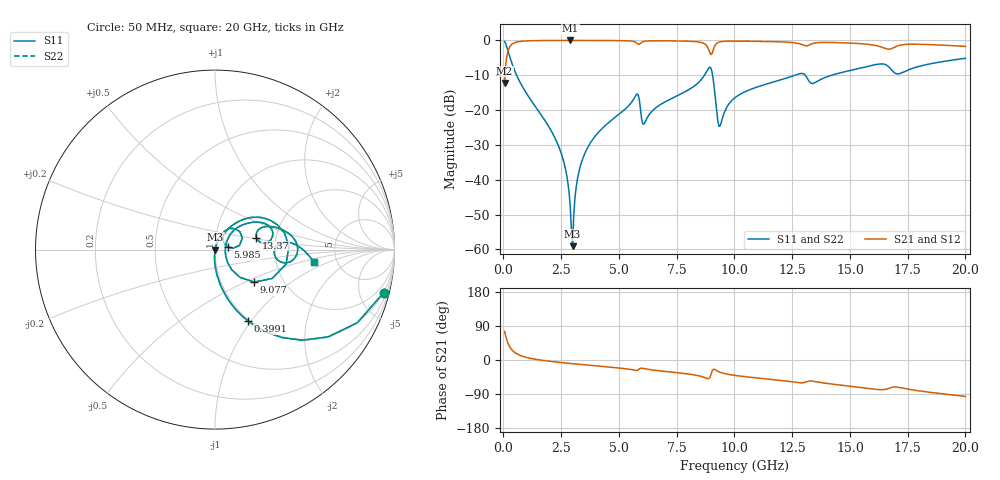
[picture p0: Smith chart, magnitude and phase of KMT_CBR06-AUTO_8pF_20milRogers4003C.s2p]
! Data measured by Modelithics Inc. support@modelithics.com 813-866-6335
! KEMET CBR06-AUTO 8pF, Pad Width= 0.851mm, Pad Length= 0.64mm, Pad Gap= 0.62mm, 20mil Rogers 4003C substrate Data, January 2022
# hz S ma R 50
! 2 Port Network Data from SP1.SP block
! freq  magS11  angS11  magS21  angS21  magS12  angS12  magS22  angS22
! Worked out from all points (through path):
!   401 points, 50 MHz to 20 GHz, reference 50 ohm
!   highest |S21| = -0.01 dB at 2.893 GHz (marker M1); lowest = -12.2 dB at 50 MHz (marker M2)
!   group delay of S21, straight-line fit = 14.5 ps
!   lowest |S11| = -59.1 dB at 2.993 GHz (marker M3), VSWR 1.00, Z = 50.1 + j0.0517 ohm
!   |S11| at or under -10 dB: 571.6 MHz to 8.702 GHz (8.13 GHz wide, 175 % of centre); 9.054 GHz to 12.62 GHz (3.561 GHz wide, 32.9 % of centre); 13.07 GHz to 14.2 GHz (1.135 GHz wide, 8.33 % of centre)
!   |S22| runs from -59.1 to -0.3 dB; largest |S21 - S12| = 0
!   S11 on the Smith chart (normalised r, x): 50 MHz: 0.98, -7.81; 399.1 MHz: 0.98, -0.96; 5.985 GHz: 1.16, +0.03; 9.077 GHz: 1.43, -0.56; 13.37 GHz: 1.58, +0.22; 20 GHz: 3.34, -0.66
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5e7  0.9693 -14.4  0.2454 75.6  0.2454 75.6  0.9693 -14.4
3.99125e8  0.4371 -65.3  0.8988 24.6  0.8988 24.6  0.4371 -65.3
2.394125e9  0.02995 -94.5  0.9987 -6.0  0.9987 -6.0  0.02995 -94.5
2.693375e9  0.01384 -94.4  0.999 -7.9  0.999 -7.9  0.01384 -94.4
2.892875e9  0.004101 -86.9  0.999 -9.1  0.999 -9.1  0.004101 -86.9
2.992625e9  0.001113 27.6  0.999 -9.7  0.999 -9.7  0.001113 27.6
3.192125e9  0.009733 73.7  0.9989 -10.9  0.9989 -10.9  0.009733 73.7
3.391625e9  0.01836 75.0  0.9988 -12.0  0.9988 -12.0  0.01836 75.0
3.990125e9  0.04299 73.2  0.9978 -15.4  0.9978 -15.4  0.04299 73.2
5.73575e9  0.163 44.8  0.9379 -27.4  0.9379 -27.4  0.163 44.8
5.985125e9  0.07381 11.2  0.9369 -21.6  0.9369 -21.6  0.07381 11.2
6.73325e9  0.1164 59.2  0.988 -28.4  0.988 -28.4  0.1164 59.2
8.678375e9  0.3075 35.7  0.9055 -45.5  0.9055 -45.5  0.3075 35.7
8.92775e9  0.4131 2.5  0.6802 -46.9  0.6802 -46.9  0.4131 2.5
9.077375e9  0.2834 -39.7  0.7231 -24.9  0.7231 -24.9  0.2834 -39.7
9.376625e9  0.05877 8.6  0.9545 -32.2  0.9545 -32.2  0.05877 8.6
1.0025e10  0.1507 45.5  0.9784 -40.7  0.9784 -40.7  0.1507 45.5
1.2818e10  0.3325 21.8  0.8959 -59.9  0.8959 -59.9  0.3325 21.8
1.336662e10  0.2405 16.1  0.8978 -55.6  0.8978 -55.6  0.2405 16.1
1.536162e10  0.3941 16.0  0.9031 -71.7  0.9031 -71.7  0.3941 16.0
1.670825e10  0.4098 -10.2  0.7492 -74.2  0.7492 -74.2  0.4098 -10.2
2e10  0.5541 -7.1  0.822 -96.1  0.822 -96.1  0.5541 -7.1
